TYPE ST_SentRxStats :
STRUCT
	nFrmRxCnt			: UDINT;
	nFrmRxCntValid		: UDINT;
	nFrmRxCntInvalid	: UDINT;
	nSlowChnCnt			: UDINT;
	nSlowChnCntValid	: UDINT;
	nSlowChnCntInvalid	: UDINT;
END_STRUCT
END_TYPE
